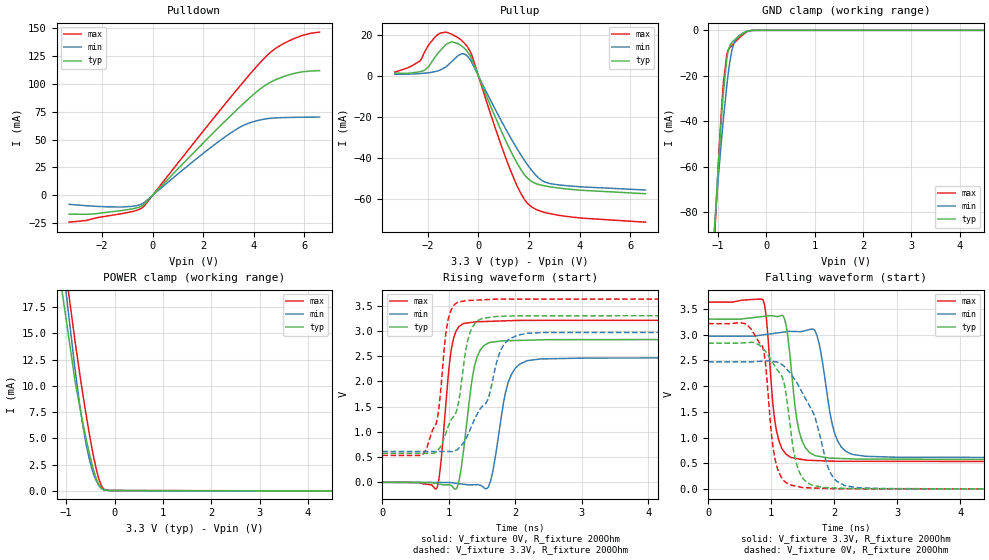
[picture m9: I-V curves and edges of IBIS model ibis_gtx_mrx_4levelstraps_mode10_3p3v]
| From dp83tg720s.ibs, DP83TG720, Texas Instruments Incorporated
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| ibis_gtx_mrx_4levelstraps_mode10_3p3v
[Model]   ibis_gtx_mrx_4levelstraps_mode10_3p3v
Model_type   I/O
Polarity   Non-Inverting
Enable   Active-Low
Vinl = 0.99
Vinh = 2.31
Vmeas = 1.65
Vref = 1.65
Cref = 2pF
Rref = 100000
|   typ   min   max
C_comp   2.49pF   2.45pF   2.54pF
[Voltage Range]   3.3   2.97   3.63
[Temperature Range]   27   150   -40
[Pullup Reference]   3.3   2.97   3.63
[Pulldown Reference]   0   0   0
[Power Clamp Reference]   3.3   2.97   3.63
[GND Clamp Reference]   0   0   0
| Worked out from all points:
|   slope of the pulldown table from 0 to 0.495 V, typ, clamps not added: 42.2 ohm
|   slope of the pullup table from 0 to 0.495 V, typ, clamps not added: 32.8 ohm
|   GND clamp passes 1 mA (typ) near -0.45 V on its own axis
|   POWER clamp passes 1 mA (typ) near -0.36 V on its own axis
|   falling waveform, V_fixture 3.3V, R_fixture 200Ohm: 20-80 % time 161ps typ, 198ps min, 136ps max; typ from 3.3 V to 0.575 V
|   rising waveform, V_fixture 0V, R_fixture 200Ohm: 20-80 % time 166ps typ, 194ps min, 132ps max; typ from 0 V to 2.83 V
|   rising waveform, V_fixture 3.3V, R_fixture 200Ohm: 20-80 % time 281ps typ, 416ps min, 155ps max; typ from 0.575 V to 3.3 V
|   falling waveform, V_fixture 0V, R_fixture 200Ohm: 20-80 % time 260ps typ, 435ps min, 157ps max; typ from 2.83 V to 0 V
[Pulldown]
|   Voltage   I(typ)   I(min)   I(max)
-3.3V     -16.77mA   -7.996mA   -24.01mA
-2.32V    -16.56mA   -9.689mA   -20.66mA
-1.211V   -13.53mA   -10.42mA   -16.37mA
-676.5mV  -11.5mA    -9.369mA   -13.77mA
-399.3mV  -9.041mA   -7.33mA    -10.9mA
2.234V    52.23mA    41.75mA    64.12mA
3.046V    70.46mA    55.28mA    86.81mA
3.59V     82.23mA    62.68mA    101.7mA
4.412V    98.01mA    68.33mA    122.8mA
4.887V    103.8mA    69.47mA    132.1mA
5.877V    110.5mA    70mA       143mA
6.6V      111.8mA    70.21mA    146.3mA
[GND Clamp]
|   Voltage   I(typ)   I(min)   I(max)
-3.3V     -1.029A    -875.3mA   -1.153A
-1.063V   -85.35mA   -85.15mA   -89.45mA
-1.053V   -81.67mA   -82.25mA   -85.19mA
-953.7mV  -47.17mA   -55.29mA   -45.08mA
-894.3mV  -29.71mA   -41.05mA   -25.54mA
-815.1mV  -12.73mA   -24.4mA    -10.64mA
-765.6mV  -7.51mA    -15.86mA   -8.098mA
-726mV    -5.811mA   -10.61mA   -7.061mA
-676.5mV  -4.664mA   -6.37mA    -5.918mA
-567.6mV  -2.714mA   -2.512mA   -3.568mA
-419.1mV  -648.2uA   -603.7uA   -953.7uA
6.6V      0A         0A         0A
[Pullup]
|   Voltage   I(typ)   I(min)   I(max)
-3.3V     1.293mA    748.4uA    1.811mA
-2.33V    1.941mA    1.084mA    7.036mA
-2.142V   2.672mA    1.267mA    11.2mA
-1.538V   11.87mA    2.646mA    20.62mA
-1.053V   16.6mA     6.952mA    20.28mA
-815.1mV  15.72mA    9.702mA    18.66mA
-537.9mV  13.21mA    10.52mA    15.72mA
-280.5mV  8.591mA    6.898mA    10.64mA
1.125V    -32.75mA   -26.9mA    -41.43mA
1.957V    -50.09mA   -43.61mA   -62.32mA
2.788V    -53.99mA   -52.36mA   -67.04mA
6.6V      -57.42mA   -55.62mA   -71.3mA
[POWER Clamp]
|   Voltage   I(typ)   I(min)   I(max)
-3.3V     318.1mA    237.2mA    400.7mA
-1.181V   22.08mA    26mA       26.9mA
-815.1mV  10.41mA    11.5mA     14.19mA
-656.7mV  6.506mA    6.277mA    9.241mA
-587.4mV  4.953mA    4.443mA    7.232mA
-528mV    3.717mA    3.154mA    5.608mA
-458.7mV  2.419mA    1.969mA    3.857mA
-369.6mV  1.074mA    887uA      1.926mA
-310.2mV  474.3uA    430.6uA    944.6uA
-231mV    113.6uA    129.2uA    222.5uA
-72.6mV   34.18uA    26.12uA    49.79uA
6.6V      0A         0A         0A
[Ramp]
R_load = 200
|   typ   min   max
dV/dt_r   1.69776/1.64854e-10   1.47976/1.9379e-10   1.92601/1.31209e-10
dV/dt_f   1.63474/1.60669e-10   1.41481/1.97861e-10   1.85696/1.3581e-10
[Falling Waveform]
V_fixture = 3.3V
V_fixture_min = 2.97V
V_fixture_max = 3.63V
R_fixture = 200Ohm
C_fixture = 0F
|   Time   V(typ)   V(min)   V(max)
0s        3.299V     2.969V     3.629V
871.5ps   3.352V     2.994V     3.671V
1.076ns   3.353V     3.028V     1.184V
1.214ns   3.294V     3.051V     712.9mV
1.313ns   2.401V     3.061V     615.7mV
1.542ns   805.9mV    3.077V     563.9mV
1.728ns   643.2mV    2.977V     554.6mV
2ns       600.3mV    1.114V     542.5mV
2.275ns   587.7mV    680.2mV    541.9mV
6ns       574.6mV    611.3mV    534.1mV
[Rising Waveform]
V_fixture = 0V
V_fixture_min = 0V
V_fixture_max = 0V
R_fixture = 200Ohm
C_fixture = 0F
|   Time   V(typ)   V(min)   V(max)
0s        134.7uV    301.4uV    79.36uV
817.9ps   -24.39mV   -2.576mV   -119.4mV
1.038ns   -66.66mV   -7.687mV   2.641V
1.129ns   -84.25mV   -22.98mV   3.039V
1.215ns   567.5mV    -37.26mV   3.141V
1.387ns   2.308V     -48.28mV   3.175V
1.601ns   2.764V     -69.13mV   3.187V
1.889ns   2.805V     1.959V     3.2V
2.165ns   2.814V     2.403V     3.207V
6ns       2.83V      2.467V     3.21V
[Rising Waveform]
V_fixture = 3.3V
V_fixture_min = 2.97V
V_fixture_max = 3.63V
R_fixture = 200Ohm
C_fixture = 0F
|   Time   V(typ)   V(min)   V(max)
0s        574.6mV    611.3mV    534.1mV
659.8ps   573.4mV    609.9mV    647mV
833.2ps   637mV      609.6mV    1.304V
988.9ps   1.101V     609.2mV    3.219V
1.143ns   1.562V     666.3mV    3.57V
1.281ns   2.795V     929.5mV    3.6V
1.388ns   3.143V     1.254V     3.607V
1.798ns   3.288V     2.661V     3.627V
2.024ns   3.297V     2.911V     3.627V
6ns       3.299V     2.969V     3.629V
[Falling Waveform]
|Gnd
V_fixture = 0V
V_fixture_min = 0V
V_fixture_max = 0V
R_fixture = 200Ohm
C_fixture = 0F
|   Time   V(typ)   V(min)   V(max)
0s        2.833V     2.47V      3.213V
579.2ps   2.841V     2.469V     3.214V
862.6ps   2.734V     2.484V     2.765V
1.06ns    2.383V     2.474V     594.2mV
1.195ns   2.111V     2.397V     177mV
1.292ns   1.328V     2.266V     85.6mV
1.511ns   196.6mV    1.834V     29.6mV
1.939ns   26.48mV    316.9mV    10.79mV
2.156ns   16.4mV     74.56mV    8.679mV
6ns       133.6uV    300.9uV    78.49uV
